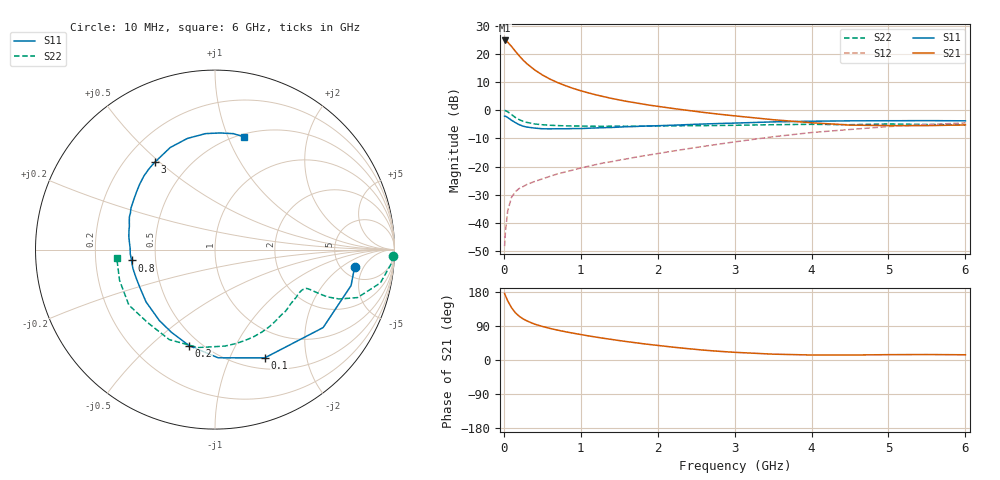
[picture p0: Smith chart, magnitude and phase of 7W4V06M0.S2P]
! Infineon Technologies  Discrete & RF Semiconductors
! BFS17W
! Si NPN RF Bipolar Junction Transistor in SOT323
! VCE = 4 V  IC = 6 mA
! Common Emitter S-Parameters:  August  1999
# GHz  S  MA  R  50
!  f  S11  S21  S12  S22
! GHz  MAG  ANG  MAG  ANG  MAG  ANG  MAG  ANG
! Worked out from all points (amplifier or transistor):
!   36 points, 10 MHz to 6 GHz, reference 50 ohm
!   highest |S21| = 24.7 dB at 10 MHz (marker M1)
!   |S21| within 3 dB of that: start of sweep to 125.7 MHz
!   unconditionally stable (mu >= 1): 512.7 MHz to 2.594 GHz; 4.475 GHz to end of sweep
!   at 250 MHz: K = 0.64, MSG = 22.4 dB, |S12| = -27.1 dB
!   at 1.4 GHz: K = 1.23, MAG = 8.3 dB, |S12| = -18.2 dB
!   at 6 GHz: K = 1.07, MAG = -2.0 dB, |S12| = -4.5 dB
!   S11 on the Smith chart (normalised r, x): 10 MHz: 6.48, -3.35; 100 MHz: 0.63, -1.36; 200 MHz: 0.43, -0.67; 800 MHz: 0.36, -0.06; 3 GHz: 0.32, +0.48; 6 GHz: 0.53, +1.14
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0.01  0.7836 -7.3  17.21 175.5  0.0039 82.8  0.9942 -2.0
0.02  0.7842 -14.8  17.09 170.1  0.0068 86.7  0.9826 -4.9
0.05  0.7428 -35.8  16.06 156.2  0.0165 75.3  0.9399 -11.4
0.1  0.6639 -65.3  13.48 138.0  0.0287 61.8  0.8382 -18.6
0.15  0.6032 -88.3  11.07 124.6  0.036 54.2  0.7439 -21.7
0.2  0.5542 -105.0  9.198 115.4  0.0411 52.2  0.6806 -22.8
0.25  0.5212 -117.6  7.743 108.5  0.0443 49.6  0.6361 -22.9
0.3  0.5026 -128.0  6.664 103.1  0.0484 49.9  0.6081 -22.9
0.4  0.4823 -142.7  5.184 94.7  0.0546 51.0  0.5708 -22.8
0.5  0.469 -153.1  4.222 88.6  0.0607 53.9  0.5529 -23.0
0.6  0.4671 -161.0  3.555 83.3  0.0674 55.1  0.5417 -23.9
0.8  0.4687 -172.6  2.725 74.6  0.0806 58.6  0.5284 -26.7
0.9  0.4727 -177.1  2.436 70.8  0.0873 60.1  0.5248 -28.3
1.1  0.4796 174.5  2.026 63.6  0.1016 61.7  0.5218 -32.3
1.3  0.4908 167.6  1.737 57.2  0.1165 63.4  0.5187 -37.0
1.6  0.5109 159.0  1.433 48.5  0.1375 65.1  0.5188 -44.2
2.2  0.5426 143.7  1.073 33.9  0.1889 67.4  0.5286 -60.6
3  0.5911 124.6  0.794 20.3  0.2748 65.6  0.5403 -84.0
3.5  0.621 113.7  0.679 15.4  0.3384 62.0  0.554 -99.7
4.5  0.6484 94.6  0.545 13.1  0.4555 50.0  0.5534 -132.7
5.5  0.6541 81.0  0.533 14.4  0.5563 37.3  0.5588 -162.1
6  0.6487 75.8  0.549 13.8  0.5954 31.0  0.5493 -175.0
